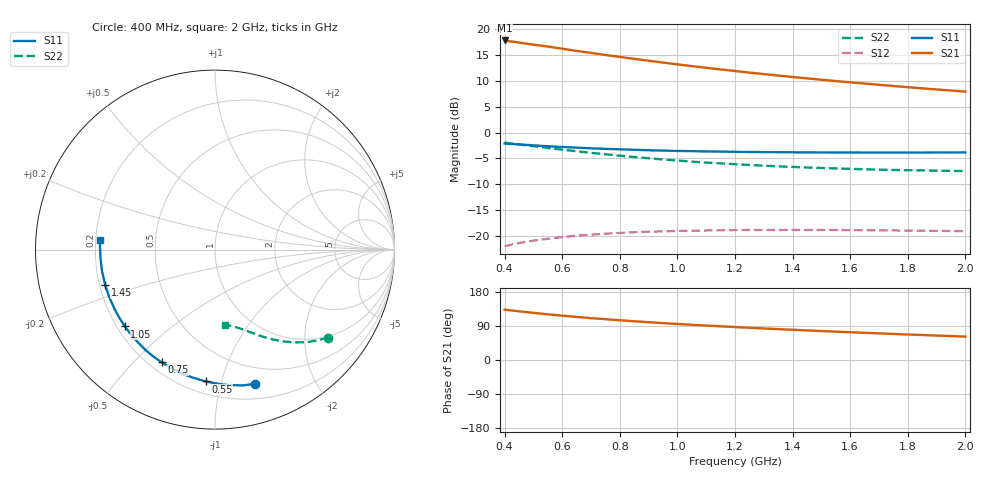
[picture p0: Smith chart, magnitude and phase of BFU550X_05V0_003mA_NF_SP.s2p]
! Filename:  P:\Prog\Test\Noise\ATS_data\Testdata_Net\BFU550X no attenuator noise\BFU550X_APG2013_44_C05_05p0V_003mA_NF_CM01_D.sf
! Date/Time: Fri 26/Jul/2013 14:37:12
! BFU550X_APG2013_44_C05_05p0V_1to10mA_NF_CM01_Bias3_R.sf
! Noise Parameter Data File
! BFU550X_APG2013_44_C05_05p0V_1to10mA_NF_CM01
! Date/time: Wed Jul 24 16:36:15 2013
! VAR V_out= 5.000000
! VAR I_out= 3.000000
! VAR V_in= 0.802000
! VAR I_in= 0.032705
! Device data file deembeded for feedlines and parallel
! Original file: \BFU550X no attenuator noise\BFU550X_APG2013_44_C05_05p0V_003mA_NF_CM01_R.sf
! Feed-files: PR005V01_100713_Feed1.s2p, PR005V01_100713_Feed2.s2p
! Parallel-file: PR005V01_100713_Par.s2p
# MHz S MA R 50
!  Freq-MHz  S11-mag  S11-arg  S21-mag  S21-arg  S12-mag  S12-arg  S22-mag  S22-arg
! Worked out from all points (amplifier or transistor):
!   37 points, 400 MHz to 2 GHz, reference 50 ohm
!   highest |S21| = 17.9 dB at 400 MHz (marker M1)
!   |S21| within 3 dB of that: start of sweep to 773.9 MHz
!   unconditionally stable (mu >= 1): nowhere
!   at 500 MHz: K = 0.19, MSG = 19.0 dB, |S12| = -21.0 dB
!   at 1.1 GHz: K = 0.41, MSG = 15.8 dB, |S12| = -19.0 dB
!   at 2 GHz: K = 0.75, MSG = 13.5 dB, |S12| = -19.1 dB
!   lowest NFmin = 0.59 dB at 420 MHz
!   S11 on the Smith chart (normalised r, x): 400 MHz: 0.33, -1.29; 550 MHz: 0.28, -0.89; 750 MHz: 0.25, -0.60; 1.05 GHz: 0.23, -0.35; 1.45 GHz: 0.22, -0.15; 2 GHz: 0.22, +0.04
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400  0.782 -73.4  7.817 132.8  0.07907 50.9  0.7996 -37.8
420  0.7745 -76.3  7.662 131.0  0.08125 49.5  0.7843 -39.2
440  0.7697 -79.3  7.544 129.3  0.08367 48.2  0.7742 -40.3
460  0.763 -82.0  7.386 127.7  0.08569 46.8  0.7626 -41.8
500  0.7508 -87.5  7.121 124.4  0.08948 44.4  0.7388 -44.0
550  0.7366 -94.0  6.818 120.5  0.09317 41.6  0.7081 -46.8
600  0.7237 -99.9  6.505 117.0  0.09676 39.1  0.6824 -49.2
650  0.7142 -105.4  6.189 113.7  0.0999 36.9  0.659 -51.4
700  0.7032 -110.7  5.921 110.5  0.1022 34.7  0.6354 -53.5
750  0.6949 -115.4  5.646 107.7  0.1045 33.0  0.6158 -55.3
800  0.6874 -120.1  5.413 104.9  0.1062 31.2  0.5959 -57.1
850  0.6806 -124.5  5.182 102.2  0.1079 29.6  0.5791 -58.7
900  0.6731 -128.7  4.971 99.7  0.1092 28.1  0.5636 -60.2
950  0.6685 -132.5  4.77 97.3  0.11 26.8  0.5477 -61.8
1050  0.6599 -139.5  4.408 92.9  0.1114 24.6  0.5219 -64.4
1100  0.656 -142.8  4.242 90.9  0.1122 23.5  0.5112 -65.6
1200  0.6505 -149.0  3.95 86.9  0.1131 21.7  0.4926 -67.9
1300  0.6462 -154.6  3.69 83.2  0.1134 20.2  0.477 -70.0
1450  0.6423 -162.2  3.352 78.1  0.1135 18.4  0.4582 -73.0
1500  0.6412 -164.6  3.25 76.4  0.1135 17.9  0.453 -73.9
1750  0.6396 -175.3  2.827 68.8  0.1123 16.1  0.4336 -78.5
2000  0.642 175.5  2.495 61.8  0.1106 15.5  0.4233 -82.7
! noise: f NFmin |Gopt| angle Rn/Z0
400  0.6096  0.3247  32.45  0.15
460  0.6021  0.3049  43.25  0.1209
600  0.6732  0.3332  52.94  0.14
800  0.6912  0.344  70.89  0.1173
1000  0.7544  0.3641  85.78  0.1082
1200  0.795  0.3744  102.5  0.0981
1400  0.8666  0.4044  115  0.0888
1600  0.8171  0.4253  132.4  0.0673
1800  0.8538  0.4476  145.7  0.0561
2000  0.9293  0.4262  158.9  0.0593
